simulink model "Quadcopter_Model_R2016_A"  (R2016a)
settings: Solver=VariableStepAuto  SolverMode=SingleTasking  StartTime=0.0  StopTime=10.0  RelTol=1e-3
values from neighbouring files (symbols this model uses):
  g = 9.81    [modelParameters.m]    (also in getMomentOfInertia.m = 9.80665)
  If = 0.511    [modelParameters.m]    (also in thrustDragConstantCalculations.m = [If0; If1; If2; If3]; Kd_error.m = I_0 * sign(rotor_speed_0) + I_1 * rotor_speed_0 + I_2 * roto)
  Jreq = 4.2012e-05    [modelParameters.m]
  Jxx = 0.0218    [modelParameters.m]
  Jyy = 0.0277    [modelParameters.m]
  Jzz = 0.0332    [modelParameters.m]
  Kd = 1.8087e-07    [modelParameters.m]    (also in calcDragConstant.m = ((A'*A)^-1)*A'*b; thrustDragConstantCalculations.m = calcDragConstant(data, Pmin, Pmax, Rm, Kv, Kq, If ))
  Kq = 96.3422    [modelParameters.m]    (also in thrustDragConstantCalculations.m; Kd_error.m)
  Kt = 8.1558*10^-6    (= 8.1558e-06)    [modelParameters.m]    (also in calcThrustConstant.m = ((A'*A)^(-1))*(A'*T); thrustDragConstantCalculations.m = calcThrustConstant(data))
  Kv = 96.3422    [modelParameters.m]    (also in thrustDragConstantCalculations.m; Kd_error.m)
  m = 1.19    [modelParameters.m]
  Pmax = 0.80    (= 0.8)    [modelParameters.m]    (also in thrustDragConstantCalculations.m; Kd_error.m)
  Pmin = 0.40    (= 0.4)    [modelParameters.m]    (also in thrustDragConstantCalculations.m; Kd_error.m)
  rhx = 0.016    [modelParameters.m]
  rhy = 0.016    [modelParameters.m]
  rhz = 0.003    [modelParameters.m]
  Rm = 0.2308    [modelParameters.m]    (also in thrustDragConstantCalculations.m; Kd_error.m)
  Vb = 11.1    [modelParameters.m]    (also in calcDragConstant.m = [data.(6); data.(6); data.(6); data.(6)]; Kd_error.m = data.(6))
libraries: simulink x6

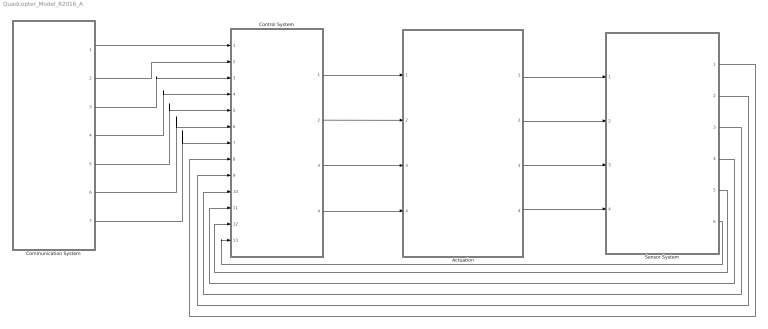
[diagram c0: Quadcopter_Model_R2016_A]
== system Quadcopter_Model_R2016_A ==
  Actuation : Subsystem
  Communication System : Subsystem
  Control System : Subsystem
  Sensor System : Subsystem
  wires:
  Control System/1(Rotor 0 Duty Cycle) -> Actuation/1(Rotor 0 Duty Cycle)
  Sensor System/6(Yaw rate (psi dot)) -> Control System/13(Yaw rate (psi dot))
  Sensor System/5(Roll rate (theta dot)) -> Control System/12(Roll rate (theta dot))
  Sensor System/4(Pitch rate (phi dot)) -> Control System/11(Pitch rate (phi dot))
  Sensor System/3(Yaw (psi)) -> Control System/10(Yaw (psi))
  Sensor System/2(Roll (theta)) -> Control System/9(Roll (theta))
  Sensor System/1(Pitch (phi)) -> Control System/8(Pitch (phi))
  Communication System/1(x_position) -> Control System/1(x position)
  Communication System/2(y_position) -> Control System/2(y position)
  Communication System/3(z_position) -> Control System/3(z position)
  Communication System/4(x_setpoint) -> Control System/4(x setpoint)
  Communication System/5(y_setpoint) -> Control System/5(y setpoint)
  Communication System/6(z_setpoint) -> Control System/6(z setpoint)
  Communication System/7(yaw_setpoint) -> Control System/7("Yaw setpoint ")
  Control System/2(Rotor 1 Duty Cycle) -> Actuation/2(Rotor 1 Duty Cycle)
  Control System/3(Rotor 2 Duty Cycle) -> Actuation/3(Rotor 2 Duty Cycle)
  Control System/4(Rotor 3 Duty Cycle) -> Actuation/4(Rotor 3 Duty Cycle)
  Actuation/1(B_omega) -> Sensor System/1(B_omega)
  Actuation/2(euler_angles) -> Sensor System/2(euler_angles)
  Actuation/3(B_vo) -> Sensor System/3(B_vo)
  Actuation/4(E_ro) -> Sensor System/4(E_ro)

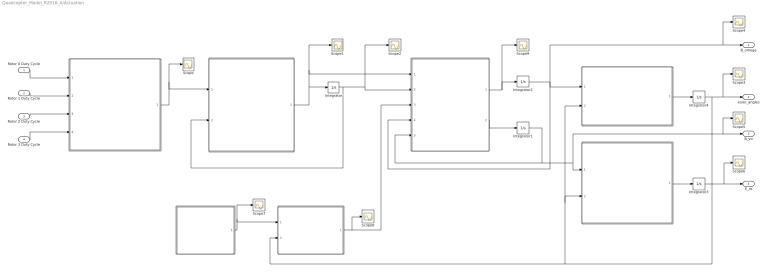
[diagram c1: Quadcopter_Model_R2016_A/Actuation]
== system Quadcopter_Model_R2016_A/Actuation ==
  Rotor 0 Duty Cycle : Inport
  Rotor 1 Duty Cycle : Inport  Port=2
  Rotor 2 Duty Cycle : Inport  Port=3
  Rotor 3 Duty Cycle : Inport  Port=4
  " " : MATLAB Function  TreatAsAtomicUnit=on
  " " : MATLAB Function  TreatAsAtomicUnit=on
  " " : MATLAB Function  TreatAsAtomicUnit=on
  " " : MATLAB Function  TreatAsAtomicUnit=on
  " " : MATLAB Function  TreatAsAtomicUnit=on
  " " : MATLAB Function  TreatAsAtomicUnit=on
  " " : MATLAB Function  TreatAsAtomicUnit=on
  Integrator{,1..3} (4 alike) : Integrator
  Integrator4 : Integrator  ContinuousStateAttributes=['phi' 'theta' 'psi']
  Scope{,1..9} (10 alike) : Scope
  B_omega : Outport
  euler_angles : Outport  Port=2
  B_vo : Outport  Port=3
  E_ro : Outport  Port=4
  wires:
  Rotor 3 Duty Cycle/1 -> " "/4(rotor_3_duty_cycle)
  Rotor 2 Duty Cycle/1 -> " "/3(rotor_2_duty_cycle)
  Rotor 1 Duty Cycle/1 -> " "/2(rotor_1_duty_cycle)
  Rotor 0 Duty Cycle/1 -> " "/1(rotor_0_duty_cycle)
  " "/1(Vb_eff) -> Scope/1, " "/1(Vb_eff)
  " "/1(angular_acceleration) -> Integrator/1, Scope1/1, " "/1(angular_acceleration)
  Integrator/1 -> Scope2/1, " "/2(angular_velocity), " "/2(angular_velocity)
  " "/1(B_omega_dot) -> Scope9/1, Integrator2/1
  " "/2(B_vo_dot) -> Integrator1/1
  Integrator2/1 -> Scope4/1, B_omega/1, " "/4(B_omega), " "/1(B_omega)
  Integrator1/1 -> " "/5(B_vo), " "/1(B_vo), B_vo/1, Scope5/1
  " "/1(euler_rates) -> Integrator4/1
  Integrator4/1 -> Scope3/1, euler_angles/1, " "/2(euler_angles), " "/2(euler_angles), " "/2(euler_angles)
  " "/1(E_Fg) -> Scope7/1, " "/1(E_Fg)
  " "/1(E_ro) -> Integrator3/1
  Integrator3/1 -> Scope6/1, E_ro/1
  " "/1(B_Fg) -> Scope8/1, " "/3(B_Fg)

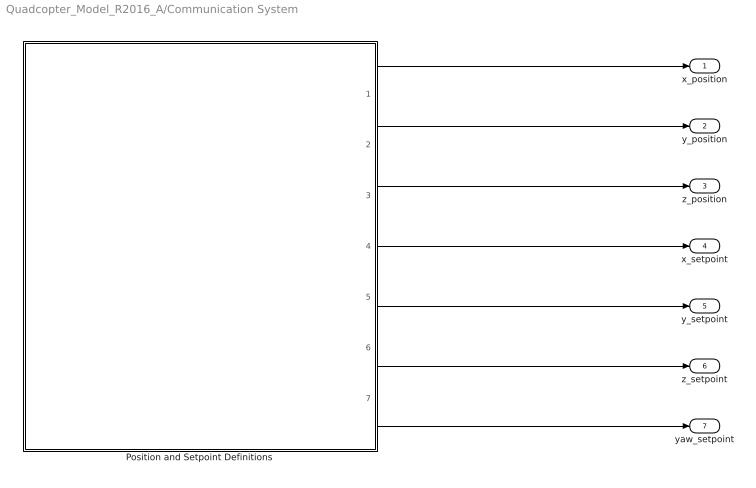
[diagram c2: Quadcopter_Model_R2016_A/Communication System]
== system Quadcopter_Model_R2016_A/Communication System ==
  Position and Setpoint Definitions : MATLAB Function  TreatAsAtomicUnit=on
  x_position : Outport
  y_position : Outport  Port=2
  z_position : Outport  Port=3
  x_setpoint : Outport  Port=4
  y_setpoint : Outport  Port=5
  z_setpoint : Outport  Port=6
  yaw_setpoint : Outport  Port=7
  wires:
  Position and Setpoint Definitions/7(yaw_setpoint) -> yaw_setpoint/1
  Position and Setpoint Definitions/6(z_setpoint) -> z_setpoint/1
  Position and Setpoint Definitions/5(y_setpoint) -> y_setpoint/1
  Position and Setpoint Definitions/4(x_setpoint) -> x_setpoint/1
  Position and Setpoint Definitions/3(z_position) -> z_position/1
  Position and Setpoint Definitions/2(y_position) -> y_position/1
  Position and Setpoint Definitions/1(x_position) -> x_position/1

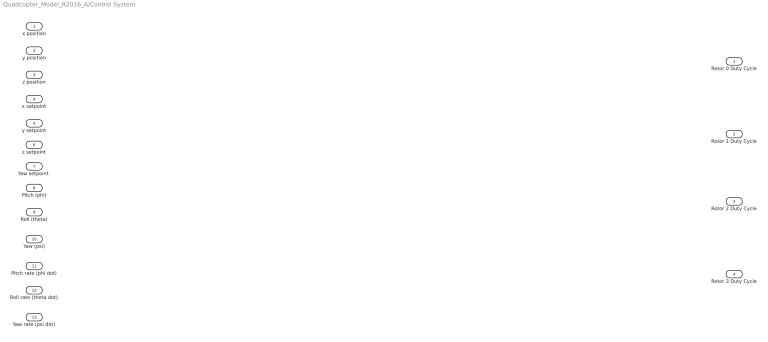
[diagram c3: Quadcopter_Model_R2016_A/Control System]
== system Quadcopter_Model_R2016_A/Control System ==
  x position : Inport
  y position : Inport  Port=2
  z position : Inport  Port=3
  x setpoint : Inport  Port=4
  y setpoint : Inport  Port=5
  z setpoint : Inport  Port=6
  "Yaw setpoint " : Inport  Port=7
  Pitch (phi) : Inport  Port=8
  Roll (theta) : Inport  Port=9
  Yaw (psi) : Inport  Port=10
  Pitch rate (phi dot) : Inport  Port=11
  Roll rate (theta dot) : Inport  Port=12
  Yaw rate (psi dot) : Inport  Port=13
  Rotor 0 Duty Cycle : Outport
  Rotor 1 Duty Cycle : Outport  Port=2
  Rotor 2 Duty Cycle : Outport  Port=3
  Rotor 3 Duty Cycle : Outport  Port=4

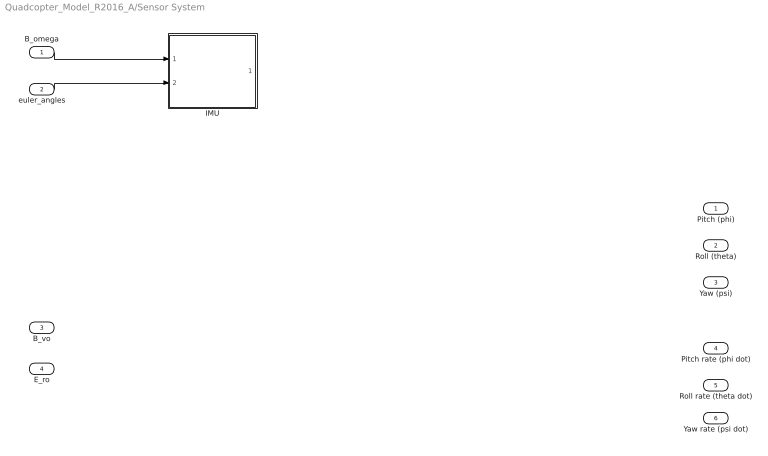
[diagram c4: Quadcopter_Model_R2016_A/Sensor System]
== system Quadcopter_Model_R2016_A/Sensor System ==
  B_omega : Inport
  euler_angles : Inport  Port=2
  B_vo : Inport  Port=3
  E_ro : Inport  Port=4
  IMU : Subsystem
  Pitch (phi) : Outport
  Roll (theta) : Outport  Port=2
  Yaw (psi) : Outport  Port=3
  Pitch rate (phi dot) : Outport  Port=4
  Roll rate (theta dot) : Outport  Port=5
  Yaw rate (psi dot) : Outport  Port=6
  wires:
  B_omega/1 -> IMU/1(B_omega)
  euler_angles/1 -> IMU/2(euler_angles)

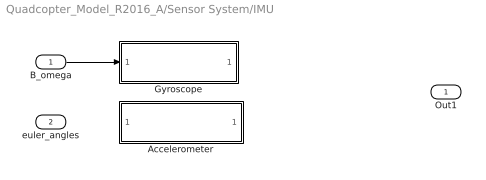
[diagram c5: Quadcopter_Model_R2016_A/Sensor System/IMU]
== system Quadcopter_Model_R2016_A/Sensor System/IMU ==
  B_omega : Inport
  euler_angles : Inport  Port=2
  Accelerometer : Subsystem
  Gyroscope : Subsystem
  Out1 : Outport
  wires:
  B_omega/1 -> Gyroscope/1(B_omega)

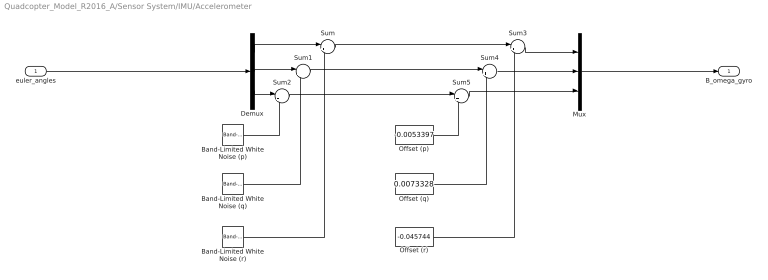
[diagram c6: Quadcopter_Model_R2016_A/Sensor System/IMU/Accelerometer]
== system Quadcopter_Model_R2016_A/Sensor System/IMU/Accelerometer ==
  euler_angles : Inport
  Band-Limited White Noise (p) : simulink/Sources/Band-Limited White Noise  Cov=[0.1]  Ts=0.1  seed=[23341]
  Band-Limited White Noise (q) : simulink/Sources/Band-Limited White Noise  Cov=[0.1]  Ts=0.1  seed=[23341]
  Band-Limited White Noise (r) : simulink/Sources/Band-Limited White Noise  Cov=[0.1]  Ts=0.1  seed=[23341]
  Demux : Demux  Outputs=3
  Mux : Mux  Inputs=3
  Offset (p) : Constant  Value=-0.0053397
  Offset (q) : Constant  Value=0.0073328
  Offset (r) : Constant  Value=-0.045744
  Sum{,1..5} (6 alike) : Sum  Inputs=|++
  B_omega_gyro : Outport
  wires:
  Demux/1 -> Sum/1
  Demux/2 -> Sum1/1
  Demux/3 -> Sum2/1
  Band-Limited White Noise (p)/1 -> Sum2/2
  Band-Limited White Noise (q)/1 -> Sum1/2
  Band-Limited White Noise (r)/1 -> Sum/2
  Sum2/1 -> Sum5/1
  Sum1/1 -> Sum4/1
  Sum/1 -> Sum3/1
  Offset (p)/1 -> Sum5/2
  Offset (r)/1 -> Sum3/2
  Offset (q)/1 -> Sum4/2
  Sum3/1 -> Mux/1
  Sum4/1 -> Mux/2
  Sum5/1 -> Mux/3
  Mux/1 -> B_omega_gyro/1
  euler_angles/1 -> Demux/1

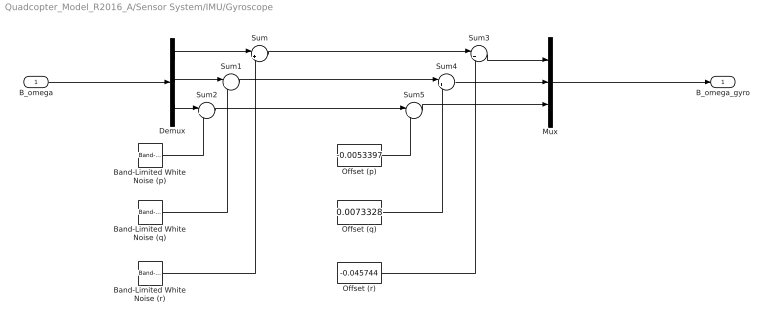
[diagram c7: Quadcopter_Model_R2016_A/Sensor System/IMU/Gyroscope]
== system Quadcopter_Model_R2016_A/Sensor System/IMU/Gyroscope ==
  B_omega : Inport
  Band-Limited White Noise (p) : simulink/Sources/Band-Limited White Noise  Cov=[0.1]  Ts=0.1  seed=[23341]
  Band-Limited White Noise (q) : simulink/Sources/Band-Limited White Noise  Cov=[0.1]  Ts=0.1  seed=[23341]
  Band-Limited White Noise (r) : simulink/Sources/Band-Limited White Noise  Cov=[0.1]  Ts=0.1  seed=[23341]
  Demux : Demux  Outputs=3
  Mux : Mux  Inputs=3
  Offset (p) : Constant  Value=-0.0053397
  Offset (q) : Constant  Value=0.0073328
  Offset (r) : Constant  Value=-0.045744
  Sum{,1..5} (6 alike) : Sum  Inputs=|++
  B_omega_gyro : Outport
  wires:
  Demux/1 -> Sum/1
  Demux/2 -> Sum1/1
  Demux/3 -> Sum2/1
  B_omega/1 -> Demux/1
  Band-Limited White Noise (p)/1 -> Sum2/2
  Band-Limited White Noise (q)/1 -> Sum1/2
  Band-Limited White Noise (r)/1 -> Sum/2
  Sum2/1 -> Sum5/1
  Sum1/1 -> Sum4/1
  Sum/1 -> Sum3/1
  Offset (p)/1 -> Sum5/2
  Offset (r)/1 -> Sum3/2
  Offset (q)/1 -> Sum4/2
  Sum3/1 -> Mux/1
  Sum4/1 -> Mux/2
  Sum5/1 -> Mux/3
  Mux/1 -> B_omega_gyro/1

== matlab function Quadcopter_Model_R2016_A/Actuation/



 ==
function E_Fg = gravity(  m, g)

E_Fg = [0; 0; m*g];

== matlab function Quadcopter_Model_R2016_A/Actuation/






 ==
function E_ro  = linear_body_earth_conversion(B_vo, euler_angles)

euler_rates = zeros(3,1);
E_ro = zeros(3,1);

phi = euler_angles(1);
theta = euler_angles(2);
psi = euler_angles(3);

Leb = [cos(theta)*cos(psi), sin(phi)*sin(theta)*cos(psi)-cos(phi)*sin(psi), cos(phi)*sin(theta)*cos(psi)+sin(phi)*sin(psi); ...
       cos(theta)*sin(psi), sin(phi)*sin(theta)*sin(psi)+cos(phi)*cos(psi), cos(phi)*sin(theta)*sin(psi)-sin(phi)*cos(psi); ...
           -sin(theta)    ,                sin(phi)*cos(theta)            ,                 cos(phi)*cos(theta)           ];

E_ro = Leb * B_vo;

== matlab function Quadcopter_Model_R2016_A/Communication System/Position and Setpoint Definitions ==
function [x_position, y_position, z_position, x_setpoint,...
    y_setpoint, z_setpoint, yaw_setpoint]= positionAndSetpointDefinitions

x_position = 0;
y_position = 0;
z_position = 0;
x_setpoint = 0;
y_setpoint = 0;
z_setpoint = 0;
yaw_setpoint = 0;

end

== matlab function Quadcopter_Model_R2016_A/Actuation/

 ==
function Vb_eff   = ESC(rotor_0_duty_cycle, rotor_1_duty_cycle, rotor_2_duty_cycle, rotor_3_duty_cycle, Pmin, Pmax, Vb)

% Define u_Pi for each of the rotors
u_P0 = (rotor_0_duty_cycle/100 - Pmin) / (Pmax - Pmin);
u_P1 = (rotor_1_duty_cycle/100 - Pmin) / (Pmax - Pmin);
u_P2 = (rotor_2_duty_cycle/100 - Pmin) / (Pmax - Pmin);
u_P3 = (rotor_3_duty_cycle/100 - Pmin) / (Pmax - Pmin);

% Determine the effective battery voltage from each ESC
Vb_eff_0 = u_P0 * Vb;
Vb_eff_1 = u_P1 * Vb;
Vb_eff_2 = u_P2 * Vb;
Vb_eff_3 = u_P3 * Vb;

Vb_eff = [Vb_eff_0, Vb_eff_1, Vb_eff_2, Vb_eff_3];

== matlab function Quadcopter_Model_R2016_A/Actuation/
 ==
function angular_acceleration  = motor(Vb_eff, angular_velocity, Rm, Kv, Kq, Kd, If, Jreq)

angular_acceleration = zeros(1,4);

% Define each motors effective battery voltage
Vb_eff_0 = Vb_eff(1);
Vb_eff_1 = Vb_eff(2);
Vb_eff_2 = Vb_eff(3);
Vb_eff_3 = Vb_eff(4);

% Determine the angular velocity of each rotor from feedback
w_0 = angular_velocity(1);
w_1 = angular_velocity(2);
w_2 = angular_velocity(3);
w_3 = angular_velocity(4);

% Determine angular acceleration of each rotor
w_0_dot = 1/(Jreq*Rm*Kq) * Vb_eff_0 - 1/(Jreq*Rm*Kq*Kv) * w_0 - 1/(Jreq*Kq)*If - (Kd/Jreq) * w_0^2;
w_1_dot = 1/(Jreq*Rm*Kq) * Vb_eff_1 - 1/(Jreq*Rm*Kq*Kv) * w_1 - 1/(Jreq*Kq)*If - (Kd/Jreq) * w_1^2;
w_2_dot = 1/(Jreq*Rm*Kq) * Vb_eff_2 - 1/(Jreq*Rm*Kq*Kv) * w_2 - 1/(Jreq*Kq)*If - (Kd/Jreq) * w_2^2;
w_3_dot = 1/(Jreq*Rm*Kq) * Vb_eff_3 - 1/(Jreq*Rm*Kq*Kv) * w_3 - 1/(Jreq*Kq)*If - (Kd/Jreq) * w_3^2;

angular_acceleration = [w_0_dot, w_1_dot, w_2_dot, w_3_dot];

== matlab function Quadcopter_Model_R2016_A/Actuation/







 ==
function [B_omega_dot, B_vo_dot]= rotor(angular_acceleration, angular_velocity, B_Fg, B_omega, B_vo, m, Kt, Kd, rhx, rhy, rhz, Jreq, Jxx, Jyy, Jzz)

B_vo_dot = zeros(3,1);
B_omega_dot = zeros(3,1);

% Create J vector
J = [Jxx,  0 ,  0 ; ...
      0 , Jyy,  0 ; ...
      0 ,  0 , Jzz;];

% Create r_hi vector
rh_0 = [-rhx; rhy; rhz];
rh_1 = [rhx; rhy; rhz];
rh_2 = [-rhx; -rhy; rhz];
rh_3 = [rhx; -rhy; rhz];

% Define vector from body frame origin to center of mass
br_oc = [0; 0; 0];

% Define 3x3 Identity Matrix
I = eye(3);

% Create gamma vectors
gamma_Ti = [0; 0; -1];
gamma_omega_03 = [0; 0; -1];  %Rotors 0 and 3 use this gamma_omega vector
gamma_omega_12 = [0; 0; 1]; %Rotors 1 and 2 use this gamma_omega vector

% Define angular velocities for each rotor
w_0 = angular_velocity(1);
w_1 = angular_velocity(2);
w_2 = angular_velocity(3);
w_3 = angular_velocity(4);

% Define angular acceleration for each rotor
w_0_dot = angular_acceleration(1);
w_1_dot = angular_acceleration(2);
w_2_dot = angular_acceleration(3);
w_3_dot = angular_acceleration(4);

% Define the rotor force in the z-direction from each rotor
B_Fr_0 = Kt * w_0 * w_0 * gamma_Ti;
B_Fr_1 = Kt * w_1 * w_1 * gamma_Ti;
B_Fr_2 = Kt * w_2 * w_2 * gamma_Ti;
B_Fr_3 = Kt * w_3 * w_3 * gamma_Ti;

% Sum up the rotor forces in the z-direction from each vector to get the
% total body force in the z-direction
B_Fr = B_Fr_0 + B_Fr_1 + B_Fr_2 + B_Fr_3;

% Define the in-plane drag and induced torque produced by each rotor
 B_Q_d0 = -1 * Kd * w_0 * w_0 * gamma_omega_03;
 B_Q_d1 = -1 * Kd * w_1 * w_1 * gamma_omega_12;
 B_Q_d2 = -1 * Kd * w_2 * w_2 * gamma_omega_12;
 B_Q_d3 = -1 * Kd * w_3 * w_3 * gamma_omega_03;

% Sum up the total in-plane drag and induced torque to get the total
% in-plane drag and induced torque on the body
B_Q_d = B_Q_d0 + B_Q_d1 + B_Q_d2 + B_Q_d3;

% Define the force lever arm torque created from the force produced by each
% rotor in the z-direction
B_Q_F0 = cross( rh_0, B_Fr_0 );
B_Q_F1 = cross( rh_1, B_Fr_1 );
B_Q_F2 = cross( rh_2, B_Fr_2 );
B_Q_F3 = cross( rh_3, B_Fr_3 );

B_Q_F = B_Q_F0 + B_Q_F1 + B_Q_F2 + B_Q_F3;

%Define the change in angular momentum torque produced by each rotor 
B_Q_L0 = -1 * Jreq * ( cross(B_omega, w_0 * gamma_omega_03) + w_0_dot * gamma_omega_03 );
B_Q_L1 = -1 * Jreq * ( cross(B_omega, w_1 * gamma_omega_12) + w_1_dot * gamma_omega_12 ); 
B_Q_L2 = -1 * Jreq * ( cross(B_omega, w_2 * gamma_omega_12) + w_2_dot * gamma_omega_12 ); 
B_Q_L3 = -1 * Jreq * ( cross(B_omega, w_3 * gamma_omega_03) + w_3_dot * gamma_omega_03 );

% Sum up the total change in angular momentum torque produced by each rotor
B_Q_L = B_Q_L0 + B_Q_L1 + B_Q_L2 + B_Q_L3;

% Define the total rotor system torque as the sum of the in-plane drag and
% induced torque, force lever arm torque, and change in angular momentum
% torques
B_Q = B_Q_d + B_Q_F + B_Q_L;

% Define the body forces in the z-direction from each vector to get the
% total body force in the z-direction
B_F = B_Fr + B_Fg; 

% Define the body frame linear velocities
B_vo_dot = (m*I)^(-1) * ( B_F - cross( B_omega, m*(B_vo + cross(B_omega, br_oc)) ) );

% Define the body frame angular velocities
B_omega_dot = J ^(-1) * ( B_Q - cross(B_omega, J * B_omega) - cross(br_oc, B_F) );

== matlab function Quadcopter_Model_R2016_A/Actuation/














 ==
function euler_rates = angular_body_earth_conversion(B_omega, euler_angles)

euler_rates = zeros(3,1);

phi = euler_angles(1);
theta = euler_angles(2);

Aeb = [1, sin(phi)*tan(theta), cos(phi)*tan(theta); ...
       0,     cos(phi)       ,        -sin(phi)   ; ...
       0,  sin(phi)/cos(theta), cos(phi)/cos(theta)];

   
euler_rates = Aeb * B_omega;

== matlab function Quadcopter_Model_R2016_A/Actuation/






















 ==
function B_Fg  = linear_earth_body_conversion(E_Fg, euler_angles)

euler_rates = zeros(3,1);
B_Fg = zeros(3,1);

phi = euler_angles(1);
theta = euler_angles(2);
psi = euler_angles(3);

Lbe = [             cos(theta)*cos(psi)              ,          cos(theta)*sin(psi)                  ,     -sin(theta)    ; ...
       sin(phi)*sin(theta)*cos(psi)-cos(phi)*sin(psi), sin(phi)*sin(theta)*sin(psi)+cos(phi)*cos(psi), sin(phi)*cos(theta); ...
       cos(phi)*sin(theta)*cos(psi)+sin(phi)*sin(psi), cos(phi)*sin(theta)*sin(psi)-sin(phi)*cos(psi), cos(phi)*cos(theta)];

B_Fg = Lbe * E_Fg;
